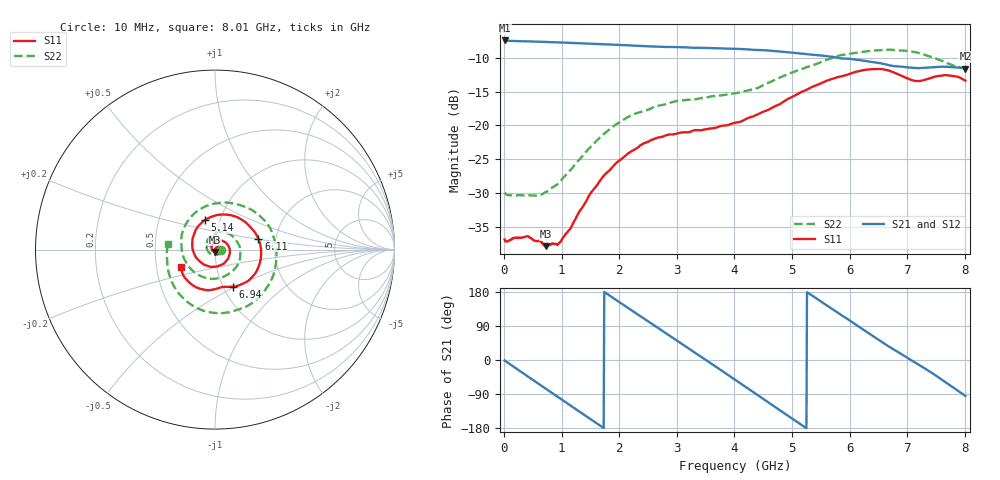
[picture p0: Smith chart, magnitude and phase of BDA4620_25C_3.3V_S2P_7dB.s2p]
!Agilent Technologies,E5071B,MY42404982,A.09.10
!Date: Wed May 06 08:49:49 2026
!Data & Calibration Information:
!Freq	S11:SOLT2(ON)	S21:SOLT2(ON)	S12:SOLT2(ON)	S22:SOLT2(ON)
# Hz S RI R 50
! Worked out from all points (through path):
!   801 points, 10 MHz to 8.01 GHz, reference 50 ohm
!   highest |S21| = -7.44 dB at 10 MHz (marker M1); lowest = -11.6 dB at 8.01 GHz (marker M2)
!   group delay of S21, straight-line fit = 283 ps
!   lowest |S11| = -37.9 dB at 720 MHz (marker M3), VSWR 1.03, Z = 50.2 - j1.27 ohm
!   |S11| at or under -10 dB: start of sweep to end of sweep
!   |S22| runs from -30.4 to -8.8 dB; largest |S21 - S12| = 0.0021
!   S11 on the Smith chart (normalised r, x): 10 MHz: 1.03, -0.00; 5.14 GHz: 0.85, +0.29; 6.11 GHz: 1.62, +0.21; 6.94 GHz: 1.11, -0.48; 8.01 GHz: 0.67, -0.14
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1e7  0.0143 -0.00083  0.4247 -0.00912  0.4251 -0.00917  0.0318 -0.00241
3.3e8  0.0131 -0.00694  0.3441 -0.2389  0.3447 -0.2396  0.0208 -0.0221
7.2e8  0.00174 -0.0126  0.1048 -0.4006  0.1049 -0.4013  -0.0121 -0.0296
9.6e8  -0.00987 -0.00915  -0.0726 -0.4041  -0.073 -0.4047  -0.0346 -0.0154
1.35e9  -0.0203 0.0134  -0.3121 -0.2576  -0.3122 -0.2579  -0.0472 0.0346
1.65e9  -0.0107 0.0364  -0.3944 -0.0607  -0.395 -0.0611  -0.0228 0.0766
1.94e9  0.0135 0.0504  -0.3685 0.1406  -0.3688 0.141  0.0269 0.0975
2.33e9  0.055 0.0415  -0.1891 0.3381  -0.1896 0.3386  0.1022 0.0703
2.68e9  0.0812 0.00568  0.0404 0.3799  0.0408 0.3801  0.1397 0.00266
3e9  0.0772 -0.0397  0.2361 0.2969  0.2367 0.2968  0.1311 -0.0758
3.39e9  0.0388 -0.0832  0.3671 0.0771  0.3674 0.0763  0.0529 -0.1486
3.69e9  -0.0093 -0.0958  0.3518 -0.1204  0.3515 -0.1214  -0.0403 -0.16
4.01e9  -0.0666 -0.0803  0.2271 -0.2899  0.2266 -0.2905  -0.1359 -0.1066
4.53e9  -0.1264 0.0156  -0.0973 -0.3455  -0.0981 -0.3461  -0.1856 0.0784
5.14e9  -0.0555 0.1655  -0.3334 -0.0668  -0.3337 -0.0663  0.00718 0.2579
5.35e9  0.00967 0.1922  -0.328 0.0581  -0.3279 0.0585  0.1071 0.2556
5.74e9  0.1469 0.1681  -0.2055 0.2448  -0.2052 0.2455  0.2759 0.1622
6.11e9  0.2415 0.0612  -0.0155 0.3062  -0.015 0.3066  0.3432 -0.0269
6.68e9  0.1873 -0.172  0.2259 0.1629  0.2269 0.1629  0.2034 -0.3
6.94e9  0.098 -0.2066  0.2651 0.0543  0.2658 0.0537  0.0643 -0.3514
7.49e9  -0.042 -0.226  0.2055 -0.1748  0.2057 -0.1758  -0.2135 -0.2293
8.01e9  -0.1908 -0.0973  -0.0219 -0.2622  -0.0222 -0.2631  -0.2619 0.0318
